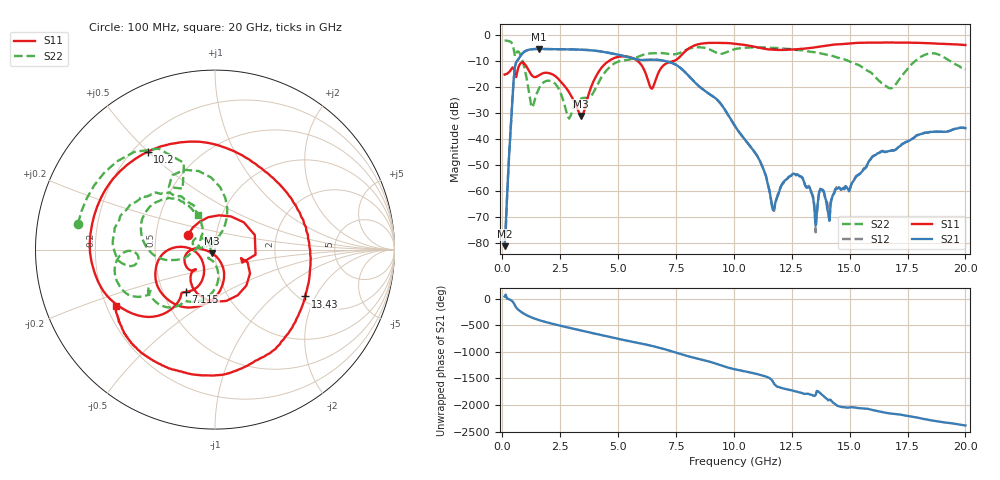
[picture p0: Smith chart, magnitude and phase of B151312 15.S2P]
!  2-Port S-parameters saved by WinCal
! VAR MeasName=S-Parameters (CALIBRATED_DATA) read from VNA (N5244A)
! VAR MeasDate=12/8/2015 5:44:41 PM
! VAR NAME=B151312 15
! VAR FILENAME=B151312 15.S2P
! VAR DATE=12/8/2015 5:44:41 PM
! VAR PHYS_PORTS=1,2
# Hz S DB R 50
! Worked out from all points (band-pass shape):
!   401 points, 100 MHz to 20 GHz, reference 50 ohm
!   highest |S21| = -5.45 dB at 1.593 GHz (marker M1); lowest = -81.4 dB at 100 MHz (marker M2)
!   |S21| within 3 dB of the highest: 765.2 MHz to 5.367 GHz (4.601 GHz wide, 150 % of centre)
!   lowest |S11| = -31.3 dB at 3.384 GHz (marker M3), VSWR 1.06, Z = 48.1 - j1.88 ohm
!   |S11| at or under -10 dB: start of sweep to 4.619 GHz; 5.83 GHz to 7.434 GHz (1.604 GHz wide, 24.2 % of centre)
!   |S22| runs from -32.3 to -2.2 dB; largest |S21 - S12| = 0.0016
!   S11 on the Smith chart (normalised r, x): 100 MHz: 0.73, +0.13; 7.115 GHz: 0.65, -0.33; 10.2 GHz: 0.26, +0.50; 13.43 GHz: 2.15, -1.65; 20 GHz: 0.24, -0.25
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1e8  -15.32 150.8  -81.39 38.4  -79.41 105.2  -2.19 169.3
5.975e8  -16.32 -18.0  -10.66 -165.9  -10.66 -165.9  -7.26 126.4
9.4575e8  -11.05 -102.4  -6.57 73.1  -6.56 73.1  -12.36 73.6
1.294e9  -15.78 -136.2  -5.56 0.7  -5.55 0.7  -27.98 125.6
1.5925e9  -15.56 -135.3  -5.45 -44.6  -5.45 -44.6  -20.50 173.9
2.5875e9  -18.66 177.2  -5.58 -158.0  -5.58 -158.0  -24.01 133.7
3.3835e9  -31.27 -134.3  -5.74 122.6  -5.74 122.6  -24.71 -129.3
3.43325e9  -31.26 -117.8  -5.76 117.7  -5.76 117.7  -24.43 -129.5
4.72675e9  -9.41 -109.1  -7.18 -8.5  -7.17 -8.6  -11.74 -97.0
5.5725e9  -8.79 -156.1  -8.92 -87.6  -8.93 -87.7  -9.39 -120.8
6.7665e9  -14.18 -112.9  -9.71 158.3  -9.71 158.3  -7.03 -144.3
7.11475e9  -10.90 -124.5  -10.28 116.8  -10.25 116.7  -7.29 -149.3
8.20925e9  -4.49 -144.8  -17.34 -23.5  -17.30 -23.6  -5.04 -155.7
1.005e10  -3.44 131.4  -35.14 111.9  -35.20 111.7  -5.51 -172.2
1.019925e10  -3.59 124.4  -37.10 98.5  -37.12 98.1  -5.27 -174.5
1.169175e10  -5.78 53.0  -67.52 -121.0  -67.22 -127.6  -5.04 161.2
1.25375e10  -5.69 11.5  -53.55 74.4  -53.66 74.4  -5.57 150.7
1.338325e10  -5.00 -25.8  -61.57 -8.0  -61.44 -13.7  -6.64 138.2
1.3433e10  -4.94 -27.4  -63.29 -22.9  -62.55 -21.6  -6.64 137.2
1.67165e10  -3.00 -113.7  -44.78 5.7  -44.53 5.4  -20.53 155.9
1.8408e10  -3.24 -137.0  -37.65 -116.7  -37.58 -116.8  -7.27 162.3
2e10  -3.94 -150.4  -35.94 138.8  -35.93 137.7  -13.34 115.7
